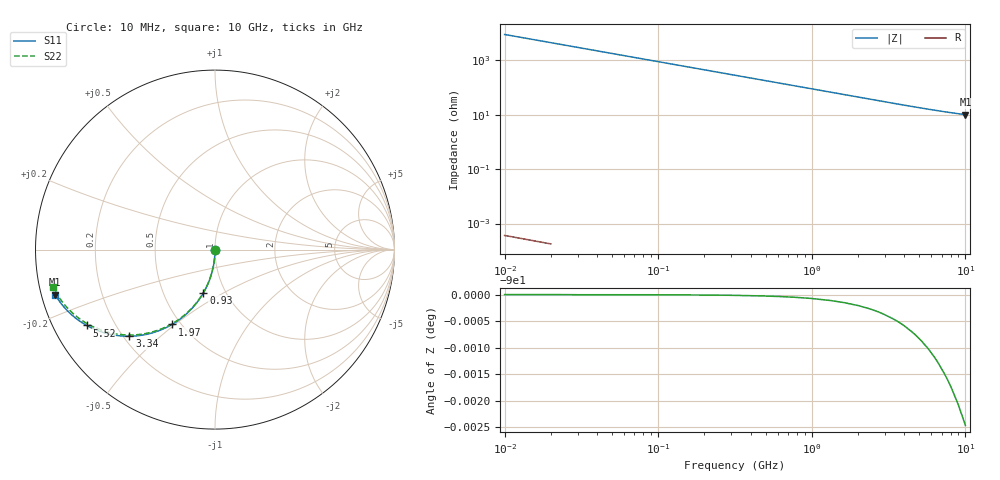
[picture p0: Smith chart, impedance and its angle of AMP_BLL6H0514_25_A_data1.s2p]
! Created Wed Apr 14 10:46:15 2010
# ghz S ma R 50
! 2 Port Network Data from SP1.SP block
! freq  magS11  angS11  magS21  angS21  magS12  angS12  magS22  angS22
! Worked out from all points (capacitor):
!   1000 points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, 10 MHz to 10 GHz, reference 50 ohm
!   read as one part in shunt: C = 1.81 pF near 60 MHz
!   lowest |Z| = 10 ohm at 10 GHz (marker M1)
!   S11 on the Smith chart (normalised r, x): 10 MHz: 1.00, -0.01; 930 MHz: 0.79, -0.41; 1.97 GHz: 0.45, -0.49; 3.34 GHz: 0.22, -0.40; 5.52 GHz: 0.10, -0.27; 10 GHz: 0.04, -0.14
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0.01  0.00278 -90.2  1 -0.2  1 -0.2  0.00278 -90.2
0.04  0.01112 -90.7  0.9999 -0.7  0.9999 -0.7  0.01112 -90.7
0.07  0.01946 -91.1  0.9998 -1.2  0.9998 -1.2  0.01946 -91.2
0.1  0.02779 -91.6  0.9996 -1.7  0.9996 -1.7  0.02779 -91.7
0.13  0.03612 -92.1  0.9993 -2.2  0.9993 -2.2  0.03612 -92.2
0.16  0.04444 -92.6  0.999 -2.7  0.999 -2.7  0.04444 -92.7
0.24  0.06659 -93.9  0.9978 -4.0  0.9978 -4.0  0.06659 -94.0
0.36  0.09962 -95.9  0.995 -6.0  0.995 -6.0  0.09962 -96.0
0.51  0.1404 -98.4  0.9901 -8.4  0.9901 -8.4  0.1404 -98.5
0.7  0.1911 -101.4  0.9816 -11.5  0.9816 -11.5  0.1911 -101.6
0.93  0.2505 -105.0  0.9681 -15.1  0.9681 -15.1  0.2505 -105.2
1.27  0.3332 -110.2  0.9429 -20.3  0.9429 -20.3  0.3332 -110.5
1.68  0.4234 -116.0  0.9059 -26.2  0.9059 -26.2  0.4234 -116.4
1.97  0.4804 -119.8  0.877 -30.1  0.877 -30.1  0.4804 -120.3
2.61  0.5866 -127.4  0.8099 -37.7  0.8099 -37.7  0.5866 -128.0
3.34  0.6783 -134.6  0.7347 -45.0  0.7347 -45.0  0.6783 -135.4
4.15  0.7517 -141.1  0.6595 -51.6  0.6595 -51.6  0.7516 -142.2
5.01  0.8062 -146.7  0.5916 -57.3  0.5916 -57.3  0.8062 -147.9
5.52  0.8305 -149.4  0.5569 -60.1  0.5569 -60.1  0.8305 -150.8
6.67  0.8704 -154.5  0.4923 -65.4  0.4923 -65.4  0.8704 -156.3
8.34  0.9053 -160.1  0.4248 -71.2  0.4248 -71.2  0.9053 -162.3
10  0.9251 -164.3  0.3796 -75.6  0.3796 -75.6  0.9251 -167.0
